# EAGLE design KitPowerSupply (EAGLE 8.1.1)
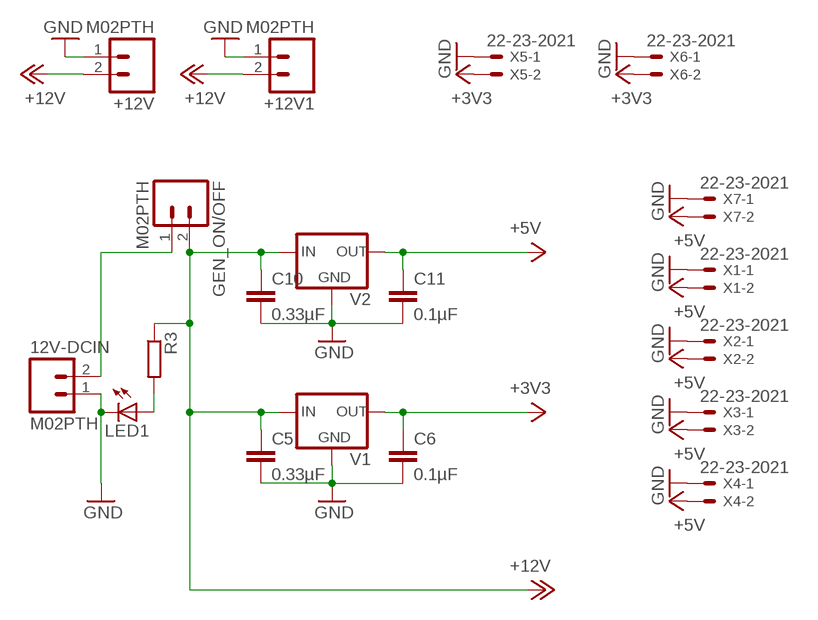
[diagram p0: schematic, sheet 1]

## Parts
12V-DCIN  M02PTH  [1X02]
+12V  M02PTH  [1X02]
+12V1  M02PTH  [1X02]
C5  0.33µF  C-EUC1206  [C1206]
C6  0.1µF  C-EUC1206  [C1206]
C10  0.33µF  C-EUC1206  [C1206]
C11  0.1µF  C-EUC1206  [C1206]
GEN_ON/OFF  M02PTH  [1X02]
LED1  LEDSMT1206  [1206]
R3  R-EU_R1206  [R1206]
V1  UA78MXX  [DPACK]
V2  UA78XX  [D2PACK]
X1  22-23-2021  [22-23-2021]
X2  22-23-2021  [22-23-2021]
X3  22-23-2021  [22-23-2021]
X4  22-23-2021  [22-23-2021]
X5  22-23-2021  [22-23-2021]
X6  22-23-2021  [22-23-2021]
X7  22-23-2021  [22-23-2021]

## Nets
+3V3: C6.1 V1.OUT X5.2 X6.2
+5V: C11.1 V2.OUT X1.2 X2.2 X3.2 X4.2 X7.2
+12V: +12V1.2 +12V.2 C5.1 C10.1 GEN_ON/OFF.2 R3.1 V1.IN V2.IN
GND: 12V-DCIN.1 +12V1.1 +12V.1 C5.2 C6.2 C10.2 C11.2 LED1.C V1.CASE(GND) V2.CASE(GND) V2.GND X1.1 X2.1 X3.1 X4.1 X5.1 X6.1 X7.1
N$1: LED1.A R3.2
N$4: 12V-DCIN.2 GEN_ON/OFF.1

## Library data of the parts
12V-DCIN +12V +12V1 GEN_ON/OFF = SparkFun-Connectors:M02: Standard 2-pin 0.1" header. Use with
C5 C6 C10 C11 = rcl:C-EU: CAPACITOR, European symbol
LED1 = led:LED: LED
R3 = rcl:R-EU_: RESISTOR, European symbol
V1 = Power:UA78MXX
V2 = Power:UA78XX
X1-X7 = con-molex:22-23-2021: .100" (2.54mm) Center Header - 2 Pin; MF: MOLEX; MPN: 22-23-2021; OC_FARNELL: 1462926; OC_NEWARK: 25C3832

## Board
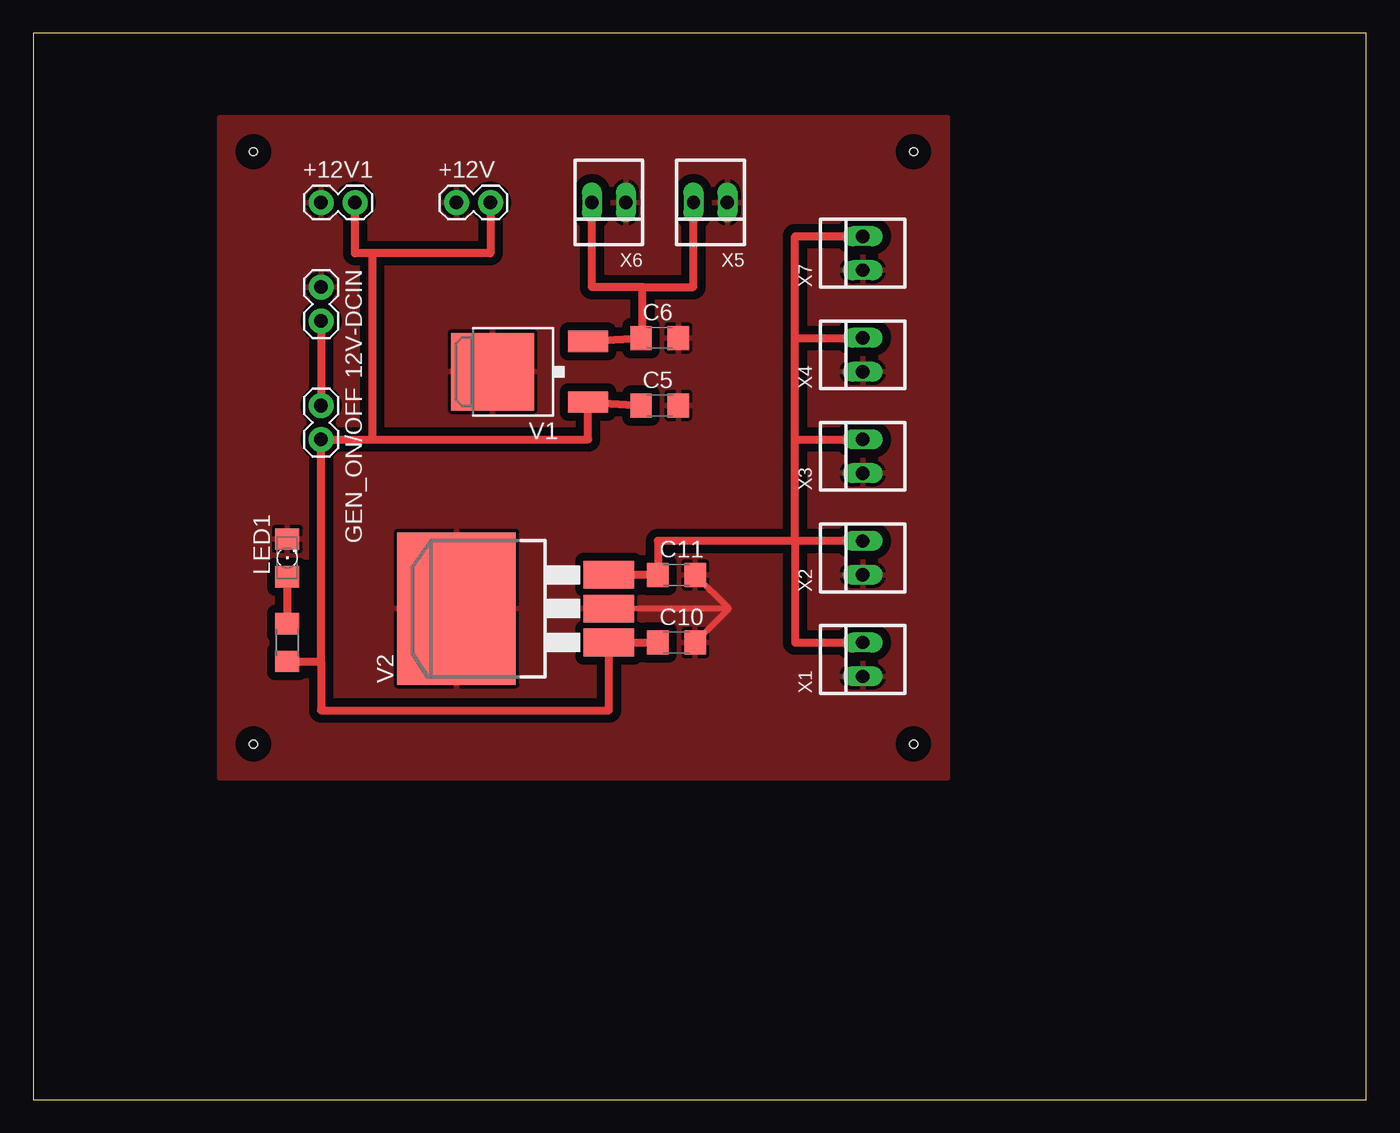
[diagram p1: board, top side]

Size 100 x 80 mm. Coordinates in mm from the lower left corner, seen from the top.
Outline: 0,0 100,0 100,80 0,80 0,0
Copper layers (1*16): Top 0.035mm / dielectric 1.5mm / Bottom 0.035mm
Design rules "default": minimum track width 10mil, minimum drill 24mil, track to track 8mil, track to pad 8mil, pad to pad 8mil, via to via 8mil, smd to smd 8mil, copper to edge 40mil, drill to drill 8mil, minimum pad ring 10mil, minimum via ring 8mil, stop-mask expansion 4mil, vias tented up to drill 0mil, thermal gap 10mil
Holes 0.6 mm at 16.51,71.12 16.51,26.67 66.04,26.67 66.04,71.12

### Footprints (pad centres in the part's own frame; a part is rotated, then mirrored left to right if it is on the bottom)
1X02 = drill 1.016 pad 1.88: 1 0,0; 2 2.54,0
C1206 = smd 1.6 x 1.8: 1 -1.4,0; 2 1.4,0
1206 = smd 1.6 x 1.803: A -1.422,0; C 1.422,0
R1206 = smd 1.6 x 1.803: 1 -1.422,0; 2 1.422,0
DPACK = smd 5.8 x 6.2: CASE 0,2.38 | smd 1.6 x 3: IN -2.28,-4.8; OUT 2.28,-4.8
D2PACK = smd 11.43 x 8.89: CASE 3.81,6.35 | smd 2.083 x 3.81: GND 3.81,-5.08; IN 1.27,-5.08; OUT 6.35,-5.08
22-23-2021 = drill 1 long: 1 -1.27,0; 2 1.27,0

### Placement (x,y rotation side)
12V-DCIN  21.59,60.96 270 top
+12V  31.75,67.31 0 top
+12V1  21.59,67.31 0 top
C5  46.99,52.07 0 top
C6  46.99,57.15 0 top
C10  48.26,34.29 0 top
C11  48.26,39.37 0 top
GEN_ON/OFF  21.59,52.07 270 top
LED1  19.05,40.64 90 top
R3  19.05,34.29 90 top
V1  36.83,54.61 90 top
V2  38.1,33.02 90 top
X1  62.23,33.02 90 top
X2  62.23,40.64 90 top
X3  62.23,48.26 90 top
X4  62.23,55.88 90 top
X5  50.8,67.31 180 top
X6  43.18,67.31 180 top
X7  62.23,63.5 90 top

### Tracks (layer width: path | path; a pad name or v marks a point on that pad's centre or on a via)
+3V3
  Top 0.406: C6.1 45.72,57.15
  Top 0.61: V1.OUT C6.1 | X6.2 41.91,60.96 45.72,60.96 | 45.72,60.96 49.53,60.96 X5.2 | 45.72,57.15 45.72,60.96
+5V
  Top 0.61: V2.OUT C11.1 46.86,41.91 57.15,41.91 | X2.2 57.15,41.91 | 57.15,41.91 57.15,49.53 | 57.15,49.53 57.15,57.15 | 57.15,57.15 X4.2 | 57.15,41.91 57.15,34.29 X1.2 | 57.15,49.53 X3.2 | 57.15,57.15 57.15,64.77 X7.2
+12V
  Top 0.61: C5.1 V1.IN 41.63,49.53 25.4,49.53 | C10.1 V2.IN 43.18,29.21 21.59,29.21 21.59,32.87 | 25.4,49.53 GEN_ON/OFF.2 21.59,32.87 | R3.1 21.59,32.87 | +12V.2 34.29,63.5 25.4,63.5 | 25.4,63.5 24.13,63.5 +12V1.2 | 25.4,63.5 25.4,49.53
GND
  Top 0.406: C11.2 52.2,36.83 | V2.GND 52.2,36.83 | 52.2,36.83 C10.2
  pour Top (isolate 0.61): 13.97,73.66 13.97,24.13 68.58,24.13 68.58,73.66
N$1
  Top 0.406: LED1.A 19.05,39.37
  Top 0.61: LED1.A R3.2
N$4
  Top 0.61: 12V-DCIN.2 GEN_ON/OFF.1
